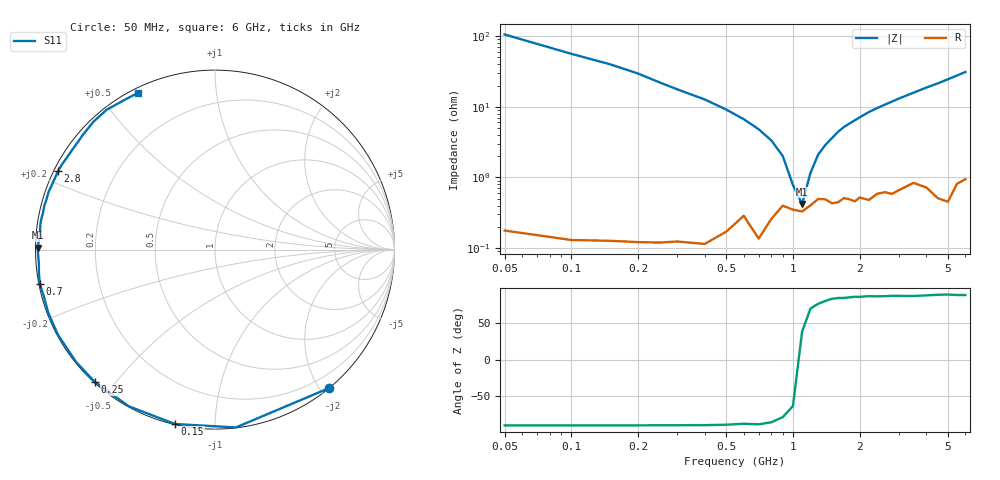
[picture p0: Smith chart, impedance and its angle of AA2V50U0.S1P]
! Infineon Technologies  Discrete & RF Semiconductors
! BBY66-02W
! Si Tuning Diode in SCD-80
! VR = 2.5 V
! S-Parameters:  June  2000
# GHz  S  MA  R  50
!  f  S11
! GHz  MAG  ANG
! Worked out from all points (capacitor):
!   34 points, 50 MHz to 6 GHz, reference 50 ohm
!   read as one part to ground: C = 28.1 pF near 50 MHz
!   lowest |Z| = 421 mohm at 1.1 GHz (marker M1)
!   series resonance near 1.073 GHz, so ESL is about 780 pH
!   S11 on the Smith chart (normalised r, x): 50 MHz: 0.00, -2.11; 150 MHz: 0.00, -0.80; 250 MHz: 0.00, -0.44; 700 MHz: 0.00, -0.10; 2.8 GHz: 0.01, +0.24; 6 GHz: 0.02, +0.62
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0.05  0.9987 -50.7
0.1  0.9977 -83.3
0.15  0.9969 -102.9
0.2  0.9964 -118.8
0.25  0.996 -132.2
0.3  0.9956 -141.0
0.4  0.9957 -151.5
0.5  0.9934 -159.3
0.6  0.9888 -164.8
0.7  0.9946 -169.0
0.8  0.9897 -172.4
1  0.9861 -178.4
1.1  0.9869 179.4
1.3  0.9804 175.3
1.5  0.983 171.8
1.6  0.9824 169.9
1.7  0.98 168.2
1.9  0.9821 165.4
2.2  0.9815 160.9
2.4  0.9775 158.3
2.8  0.9781 153.3
3  0.9756 150.8
3.5  0.97 144.9
4  0.975 139.0
4.5  0.9829 133.6
5  0.9855 127.8
5.5  0.9754 122.0
6  0.9731 116.3
